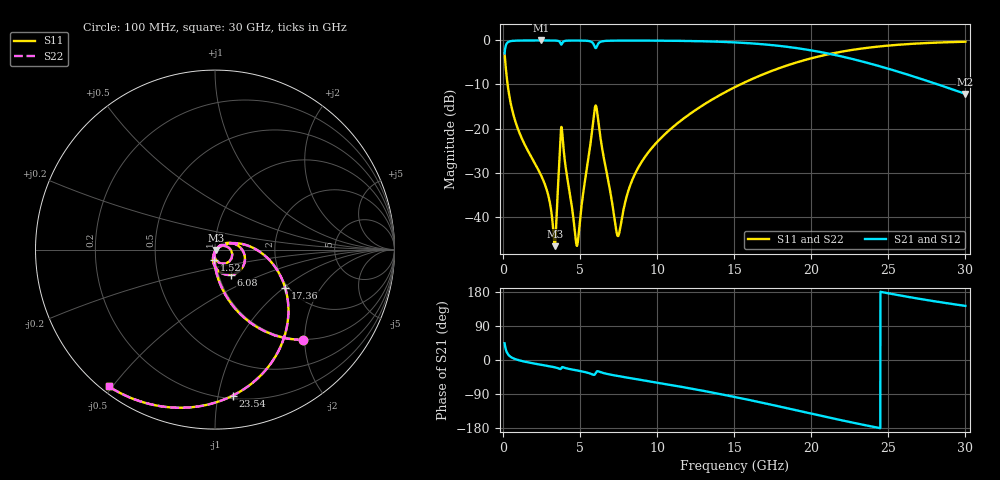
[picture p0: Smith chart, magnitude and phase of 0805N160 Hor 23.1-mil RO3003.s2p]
# GHz S MA R 50
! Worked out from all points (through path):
!   3201 points, 100 MHz to 30 GHz, reference 50 ohm
!   highest |S21| = -0.02 dB at 2.464 GHz (marker M1); lowest = -12.1 dB at 30 GHz (marker M2)
!   group delay of S21, straight-line fit = 21.5 ps
!   lowest |S11| = -46.7 dB at 3.352 GHz (marker M3), VSWR 1.01, Z = 50.4 - j0.268 ohm
!   |S11| at or under -10 dB: 295.1 MHz to 15.39 GHz (15.1 GHz wide, 192 % of centre)
!   |S22| runs from -46.7 to -0.3 dB; largest |S21 - S12| = 0
!   S11 on the Smith chart (normalised r, x): 100 MHz: 0.98, -1.95; 1.52 GHz: 0.98, -0.12; 6.08 GHz: 1.14, -0.33; 17.36 GHz: 1.93, -1.02; 23.54 GHz: 0.22, -1.10; 30 GHz: 0.02, -0.49
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0.1  0.7019 -46.0  0.7119 44.0  0.7119 44.0  0.7019 -46.0
0.436375  0.2193 -79.7  0.975 10.1  0.975 10.1  0.2193 -79.7
1.52025  0.06007 -94.1  0.9968 -5.4  0.9968 -5.4  0.06007 -94.1
2.463969  0.02955 -99.1  0.9977 -12.6  0.9977 -12.6  0.02955 -99.1
3.351625  0.004645 -34.9  0.9954 -19.3  0.9954 -19.3  0.004645 -34.9
3.46375  0.009551 24.3  0.9931 -20.4  0.9931 -20.4  0.009551 24.3
3.688  0.05896 20.1  0.9564 -23.6  0.9564 -23.6  0.05896 20.1
3.809469  0.1012 -45.8  0.9082 -19.4  0.9082 -19.4  0.1012 -45.8
4.7345  0.005148 -53.7  0.9952 -27.1  0.9952 -27.1  0.005148 -53.7
4.874656  0.005632 2.4  0.995 -28.1  0.995 -28.1  0.005632 2.4
5.089563  0.01318 34.2  0.994 -29.9  0.994 -29.9  0.01318 34.2
5.893125  0.1428 4.1  0.8913 -39.3  0.8913 -39.3  0.1428 4.1
6.08  0.1655 -58.1  0.8504 -30.3  0.8504 -30.3  0.1655 -58.1
7.453531  0.006042 -37.9  0.9937 -42.2  0.9937 -42.2  0.006042 -37.9
8.453312  0.02791 30.7  0.9944 -49.1  0.9944 -49.1  0.02791 30.7
10.06978  0.07266 25.9  0.9921 -60.2  0.9921 -60.2  0.07266 25.9
15.05  0.2954 -9.1  0.9481 -97.7  0.9481 -97.7  0.2954 -9.1
17.35791  0.4452 -28.6  0.887 -117.6  0.887 -117.6  0.4452 -28.6
20.03956  0.6288 -52.6  0.7678 -141.8  0.7678 -141.8  0.6288 -52.6
23.54347  0.8197 -83.1  0.562 -172.4  0.562 -172.4  0.8197 -83.1
25.01978  0.8734 -94.8  0.4757 175.9  0.4757 175.9  0.8734 -94.8
30  0.9655 -127.8  0.2473 142.8  0.2473 142.8  0.9655 -127.8
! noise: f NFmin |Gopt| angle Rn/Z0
0.1  0.0005848  0.8955  0.9267  0.001221
3.417  0.01038  0.8092  19.72  0.011
6.743  0.02035  0.8122  38.38  0.02019
10.06  0.01646  0.688  55.69  0.008091
13.39  0.02089  0.6855  71.76  0.008616
16.7  0.02663  0.7011  86.55  0.009503
20.03  0.03407  0.7271  100.3  0.01055
23.35  0.04412  0.7606  113.4  0.01175
26.67  0.05853  0.8002  126  0.01312
30  0.08044  0.8433  138.4  0.0144
